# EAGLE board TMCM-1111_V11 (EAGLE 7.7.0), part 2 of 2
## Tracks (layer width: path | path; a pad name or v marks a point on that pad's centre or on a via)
!4361_RST  (via drill 0.3 pad 0.8)
  Top 0.2: IC201.39 41.85,34.05 v40.55,35.35 | IC101.77 31.05,10.75 30.45,11.35 v30.05,11.35
  Bottom 0.2: v30.05,11.35 29.65,11.75 29.65,15.7 29.95,16 30.85,16 32.15,17.3 32.15,24.7 34.65,27.25 34.65,32.25 34.3,32.6 34.3,34.65 34.65,35 36.9,35 37.25,35.35 v40.55,35.35
!CS_262  (via drill 0.3 pad 0.8)
  Top 0.2: IC201.30 48.4,29.75 v48.85,30.2 | IC301.14 v51.26,26.81 v51.25,26.8
  Bottom 0.2: v51.25,26.8 48.85,29.2 v48.85,30.2
!CS_4361  (via drill 0.3 pad 0.8)
  Top 0.2: IC101.5 v32.91,13.29 v32.9,13.3 | IC201.2 39.15,29.25 v38.8,28.9
  Bottom 0.2: v32.9,13.3 v32.89,13.3 v32.9,13.29 34.31,14.7 38.6,14.7 39.45,13.85 41.25,13.85 41.7,14.3 41.7,16.2 44.8,19.3 44.8,20.15 44.1,20.85 44.1,23.25 43.75,23.6 42.5,23.6 40.7,25.4 38.6,25.4 38.15,25.85 38.15,28.25 v38.8,28.9
!CS_EEPROM  (via drill 0.3 pad 0.8)
  Top 0.2: IC503.1 10.92,4.88 v10.9,4.9 | IC101.61 22.9,9.3 v22.2,9.3
  Bottom 0.2: v10.9,4.9 15.7,4.9 16,5.2 16,6.2 18.2,8.4 21.3,8.4 v22.2,9.3
!EN_262  (via drill 0.3 pad 0.8)
  Top 0.2: IC301.15 51.71,26.31 51.45,26.05 50.7,26.05 v50.2,26.55 | IC101.75 30.05,8.35 30.5,7.9 31.5,7.9 32.1,7.3 v32.1,6
  Bottom 0.2: v32.1,6 33.15,7.05 41.45,7.05 43.5,9.1 46.1,9.1 49.85,12.85 49.85,24.7 50.5,25.35 50.5,26.25 v50.2,26.55
!INT_4361  (via drill 0.3 pad 0.8)
  Top 0.2: IC101.73 29.05,8 v31,6.05 | IC201.33 44.85,30.95 45.2,31.3 47.45,31.3 v47.75,31 | LED201.C 46.1,10.04 v46.1,10.7
  Bottom 0.2: v31,6.05 32.35,7.4 38.65,7.4 39.65,8.4 41.7,8.4 43.1,9.8 45.2,9.8 v46.1,10.7 49.15,13.75 49.15,26.4 48.15,27.4 48.15,28.15 47.7,28.6 47.7,30.95 v47.75,31
+3V3  (via drill 0.3 pad 0.8)
  Top 0.2: R501.P$6 34.1,25.4 | 34.1,25.4 33.9,25.6 33.9,26 34.1,26.2 | R501.P$7 34.1,26.2 | 34.1,26.2 33.9,26.4 33.9,26.8 34.1,27 R501.P$8 | IC503.3 13.46,4.84 12.2,6.1 IC503.7 12.19,6.09 12.1,6 11,6 10.9,6.1 10.9,7.2 IC503.8 | 34.1,25.4 33.9,25.2 33.9,24.8 34.1,24.6 R501.P$5 34.9,24.4 v35.75,24.4 | IC203.6 43.05,44.75 42.9,44.9 42.2,44.9 42.05,44.75 IC203.8 | IC201.19 45.35,24.25 45.65,23.95 v46.7,23.95 | IC201.5 40.35,27.75 39.85,27.25 38.75,27.25 38.1,27.9 38.1,28.4 C202.1 | R202.2 41.19,9.81 40.8,10.2 40.8,10.75 39.95,11.6 v39.45,11.6 | IC201.26 v47.5,27.75
  Top 0.25: IC101.50 20.09,16.29 19.9,16.1 19.49,16.1 C104.1 | IC101.70 27.55,8.25 27.9,7.9 27.9,7.45 C102.1
  Top 0.3: IC101.38 24.05,24.53 C105.1 | IC101.7 35.31,14.29 35.6,14 35.6,13.2 35.8,13 36.35,13 C106.1 | IC101.60 20.13,11.23 19.9,11 19.43,11 C103.1 | IC202.8 38.05,43.7 37.9,43.55 C209.2 | IC203.8 42.05,43.75 41.85,43.55 C212.2 | C201.1 44.85,33.35 44.25,33.35 42.85,31.95 IC201.37
  Top 0.5: v24.51,25.93 24.45,25.93 C105.1 26.13,24.93 C408.1 26.34,24.84 26.6,25.1 26.8,25.1 27.1,25.4 28.2,25.4 29.1,24.6 29.5,24.6 29.56,24.46 IC402.5 29.59,24.35 | C106.1 36.95,12.35 36.95,11.6 v37,11.6 | C104.1 18.9,15.6 18.9,15.1 v18.4,14.6 | C102.1 28.45,6.85 28.5,6.8 v28.5,6 | C103.1 19.12,10.42 19.1,10.4 v20.4,10.4 | C503.1 9.35,7.22 IC503.8 9.48,7.22 9.4,7.3 v9.4,8.3 | L101.1 39.8,20 v40.5,20 | C202.1 37.7,28.4 37.45,28.15 36.8,28.15 v36.75,28.1 | C212.2 v40.9,44.6 | C209.2 v36.9,44.6 | v43.6,33.9 44.65,33.9 C201.1 | R302.2 v62.36,25.26 v62.35,25.25 | v51.65,19.35 v47.65,19.35
  Bottom 0.5: TP4.TP 30.71,14.02 v30.7,13.2 | v43.6,33.9 44.5,34.8 44.5,43.65 43.55,44.6 v40.9,44.6 v36.9,44.6 | v62.35,25.25 61.95,25.65 59.4,25.65 57.7,23.95 53.85,23.95 51.65,21.75 v51.65,19.35
  pour Route15 (rank 3): 26.15,26.7 15.8,26.7 15.8,7.8 13.5,7.8 13.5,8.65 8.8,8.65 8.8,6.55 15.8,6.55 15.8,5.4 38.95,5.4 38.95,10.65 42.1,13.8 42.1,18.1 41.4,18.8 41.4,20.35 44.55,20.35 46.1,18.8 48.1,18.8 48.15,18.85 48.15,30.35 43.95,34.6 40.5,34.6 37.2,31.3 30.75,31.3
+5V  (via drill 0.3 pad 0.8)
  Top 0.2: R403.2 32.1,35.15 31.9,35.15 31.5,34.75 24.05,34.75 23.7,35.1 23.7,35.3 22.3,35.3 L402.2 | R503.2 16.15,7.05 15.9,7.3 15.9,8.7 15.6,9 v14.8,9 | R508.P$5 20.25,47.4 20.1,47.55 19.6,47.55 19.45,47.4 | 19.45,47.4 R508.P$6 | 18.65,47.4 18.8,47.55 19.3,47.55 19.45,47.4 | R508.P$7 18.65,47.4 | 18.65,47.4 v18.25,47.8 | 33.4,32 33.25,31.85 33.25,31.35 33.4,31.2 R201.P$8 | R201.P$6 33.4,32.8 | 33.4,32.8 33.25,32.65 33.25,32.15 33.4,32 | 33.6,33.6 33.4,33.6 33.25,33.45 33.25,32.95 33.4,32.8 | R201.P$5 33.6,33.6 | 33.6,33.6 v33.6,34.35 | R201.P$7 33.4,32 | R401.1
  Top 0.38: IC504.8 12.7,31.32 C509.1 | IC505.8 C510.1 | IC506.8 25.4,30.3 | IC204.8 50.02,43.83 49.8,43.6 48.8,43.6 48.6,43.4 C213.2
  Top 0.5: v10.97,25.83 11.87,25.83 C501.2 11.82,25.32 11.82,24.98 11.56,24.71 11.21,24.71 10.92,24.42 IC501.8 | IC502.3 13.44,9.21 C502.2 v14.8,9 | C509.1 12.65,30 12.65,30.35 12.05,30.35 11.85,30.55 11.85,30.85 v11.5,31.2 | C510.1 18.75,29.8 18.1,29.8 v17.9,29.6 | C511.1 25.4,30.3 v24.35,30.3 | 48.8,43.6 48.6,43.8 v48.6,44.6 | R401.1 41.19,18.49 41.4,18.7 41.4,18.9 v42.1,19.6
  Top 0.7: 18.75,40.2 18.79,40.25 C405.1 21,39.95 22.25,39.95 22.3,39.9 L402.2 | v20.1,38.95 19.94,38.79 D401.1 18.75,40.2 | 18.75,40.2 C406.1
  Bottom 0.5: v48.6,44.6 46.65,44.6 45.65,43.6 45.65,37.15 v48.9,33.9
  Bottom 0.7: JP401.1
  other vias: 51.7,16.9
  pour Route15 (rank 4): 56.25,0.5 4,0.5 arc-90 0.5,4 0.5,50.5 arc-90 4.5,54.5 27.5,54.5 27.5,38 46.05,38 51.55,32.5 56.2,32.5
+5V/1  (via drill 0.3 pad 0.8)
  Top 0.2: IC402.3 27.6,27.08 27.6,27.4 26.8,27.4 26.7,27.5 24.6,27.5 v24.3,27.2
  Top 0.5: C407.1 31,26.6 30.8,26.8 | 30.8,26.8 30.8,27.5 v30.6,27.7 | IC402.1 29.78,26.8 30.8,26.8 | v21.25,36.85 21.25,37.85 D401.3
  Route15 0.5: v30.6,27.7 29.95,26.95 28.1,26.95 27.45,27.6 24.75,27.6 24.35,27.2 v24.3,27.2 23.8,27.2 22.8,28.2 22.8,30.4 24.2,31.8 24.2,35.25 22.6,36.85 v21.25,36.85
/EN_D0  (via drill 0.3 pad 0.8)
  Top 0.2: IC504.1 16.57,31.43 16.6,31.4 16.6,30.9 16.7,30.8 16.7,27.7 16,27 16,25.6 16.3,25.3 16.3,24.5 15.6,23.8 v15.6,22.4 | IC101.51 22.2,15.8 v22.5,16.1
  Bottom 0.2: v22.5,16.1 20.9,17.7 20.9,21 21.1,21.2 21.1,22.2 20.6,22.7 15.9,22.7 v15.6,22.4
/EN_D1  (via drill 0.3 pad 0.8)
  Top 0.2: IC505.1 22.98,31.43 23,31.4 23,26.9 22.7,26.6 22,26.6 21.4,27.2 v17.8,27.2 | v25,15.3 24,15.3 23.6,14.9 23.2,14.9 22.09,13.79 IC101.55
  Bottom 0.2: v25,15.3 25,16.1 24.4,16.7 24.1,16.7 23.4,17.4 23.2,17.4 22.1,18.5 22.1,20.4 22.4,20.7 22.4,21.3 23.3,22.2 23.3,23 22.4,23.9 15.7,23.9 14.9,24.7 14.9,25.4 15.6,26.1 15.6,26.4 16.4,27.2 v17.8,27.2
/EN_D2  (via drill 0.3 pad 0.8)
  Top 0.2: IC506.1 29.38,31.43 29.4,31.4 29.4,29.2 29.8,28.8 v30.3,28.8 | IC101.57 22.11,12.79 22.2,12.7 23.8,12.7 v25.6,14.5
  Bottom 0.2: v30.3,28.8 30.75,28.35 31.1,28.35 31.4,28.05 31.4,27.3 30.7,26.6 29.4,26.6 29.1,26.3 29.1,18.95 28.45,18.3 28.45,16.75 27.75,16.05 27.15,16.05 v25.6,14.5
/EN_U0  (via drill 0.3 pad 0.8)
  Top 0.2: IC101.52 22.99,15.29 v23.5,15.8 | IC504.7 13.43,32.08 v13.7,31.8
  Bottom 0.2: v23.5,15.8 23.5,16.2 23.1,16.6 23,16.6 21.3,18.3 21.3,20.8 21.5,21 21.5,22.4 20.8,23.1 15.5,23.1 14.1,24.5 14.1,25.8 14.5,26.2 14.5,27.5 14,28 14,31.5 v13.7,31.8
/EN_U1  (via drill 0.3 pad 0.8)
  Top 0.2: IC505.7 19.68,32.08 20.15,31.6 v20.15,31.15 | v24.2,14.5 23.4,14.5 22.19,13.29 IC101.56
  Bottom 0.2: v24.2,14.5 24.2,16.1 23.3,17 23.1,17 21.7,18.4 21.7,20.5 22,20.8 22,21.4 22.9,22.3 22.9,22.9 22.3,23.5 15.6,23.5 14.5,24.6 14.5,25.6 15.2,26.3 15.2,26.6 16.5,27.9 18.3,27.9 20.15,29.75 v20.15,31.15
/EN_U2  (via drill 0.3 pad 0.8)
  Top 0.2: IC506.7 26.18,32.08 26.5,31.75 v26.5,31.2 | v25.9,15.8 26.35,15.35 26.35,12.15 27.1,11.4 27.1,10.8 26.55,10.25 IC101.68
  Bottom 0.2: v26.5,31.2 25.9,30.6 25.9,22.2 24.7,21 24.7,18.9 25,18.6 25,17.8 25.1,17.7 25.1,17.1 25,17 25,16.7 v25.9,15.8
AIN  (via drill 0.3 pad 0.8)
  Top 0.2: JP101.9 19.08,51.2 17.1,51.2 16.5,50.6 16.5,48.9 15,47.4 11.8,47.4 11.7,47.5 v8.4,47.5 | R502.2 10.47,30.02 10.45,30 v10.45,31.2
  Bottom 0.2: v8.4,47.5 8.4,32.2 9.4,31.2 v10.45,31.2
AIN0  (via drill 0.3 pad 0.8)
  Top 0.2: R505.2 17.15,14.1 16,14.1 14.7,12.8 | IC101.65 25.05,10.15 25.7,10.8 25.7,11.4 25.2,11.9 23.2,11.9 21,9.7 17.8,9.7 17.6,9.9 17.6,10.1 17.2,10.5 C504.1 17.2,11.1 15.9,11.1 15.1,11.9 15.1,12.4 14.7,12.8 | 14.7,12.8 v9.9,12.8 | R502.1 10.47,28.32 10.45,28.3 v10.45,27.25
  Bottom 0.2: v10.45,27.25 9.9,26.7 v9.9,12.8
AIN1
  Top 0.2: IC101.66 25.55,8.45 25.3,8.2 22.2,8.2 21.65,8.75 C505.1 R506.2 R503.1
AIN2  (via drill 0.3 pad 0.8)
  Top 0.2: IC101.67 26.05,8.15 25.4,7.5 24.95,7.5 C506.1 24.55,6.05 v24.6,6 | R504.1 35.2,42.65 R507.2 v34.1,40.3
  Bottom 0.2: v24.6,6 24.6,8.7 25.7,9.8 25.7,11.5 26,11.8 26.9,11.8 27.7,12.6 28.4,12.6 29.2,13.4 29.2,15.9 29.7,16.4 30.7,16.4 31.8,17.5 31.8,24.9 34.3,27.4 34.3,32 32.45,33.85 32.45,34.35 33.8,35.7 33.8,40 v34.1,40.3
BMA1  (via drill 0.3 pad 0.8)
  Top 0.3: 69.94,48.3 v62.1,48.3 | IC301.5 54.49,31.61 54.3,31.8 54.3,33 55,33.7 v55,34.6
  Top 0.38: X301.1 77.09,34.66 77.09,48.26 v73.91,48.26 T301.3
  Bottom 0.3: v55,34.6 56.9,36.5 56.9,44.9 59.1,47.1 60.1,47.1 61.3,48.3 v62.1,48.3
  other vias: 73.91,45.72 73.91,46.99 73.91,50.8 73.91,49.53 67.18,51.94 72.77,51.94 69.98,51.94 68.58,51.94 71.37,51.94 69.98,44.58 72.77,44.58 71.37,44.58 67.18,44.58 68.58,44.58
  pour Top (isolate 0.254, rank 3, no thermals): 66.8,43.73 66.8,54.5 81,54.5 arc-90 84.5,51 84.5,35.2 76.4,35.2 76.4,43.73
  pour Top (rank 4): 76.4,35.2 76.4,31.5 84.5,31.5 84.5,35.3 76.4,35.3
  pour Bottom: 63.5,52.96 63.5,41.66 75.18,41.66 75.18,52.96
BMA2  (via drill 0.3 pad 0.8)
  Top 0.3: 69.97,34.3 v62.1,34.3 | IC301.4 55,30.06 v55,32.5 | 70,32.9 69.98,32.92 T302.3
  Top 0.38: X301.2 77.45,30.8 70,30.8 | 79,29.2 77.8,28 70,28 70,30.8 | 70,30.8 70,32.9
  Bottom 0.3: v62.1,34.3 62.5,33.9 62.5,33 61.2,31.7 55.3,31.7 55,32 v55,32.5
  other vias: 73.91,34.29 73.91,36.83 73.91,31.75 73.91,33.02 73.91,35.56 72.77,37.97 69.98,37.97 67.18,37.97 68.58,37.97 71.37,37.97 71.37,30.61 72.77,30.61 69.98,30.61 67.18,30.61 68.58,30.61
  pour Top (rank 4, no thermals): 66.8,43.23 66.8,27.7 75.9,27.7 75.9,43.23
  pour Top (rank 4): 75.9,31.1 84.5,31.1 84.5,27.7 75.9,27.7
  pour Bottom: 63.5,41.27 63.5,27.69 75.18,27.69 75.18,41.27
BMB1  (via drill 0.3 pad 0.8)
  Top 0.3: 69.98,20.8 v62,20.8 | IC301.20 54.49,23.37 54.48,23.37 54.48,22.48 v54.1,22.1
  Top 0.38: T303.3 69.98,27 77.75,27 X301.3 77.75,24.5 70,24.5
  Bottom 0.3: v62,20.8 60.9,20.8 60.2,20.1 59.1,20.1 58.3,20.9 56.65,20.9 55.45,22.1 v54.1,22.1
  other vias: 73.91,20.83 73.91,23.37 73.91,18.29 72.77,24.51 69.98,24.51 67.18,24.51 68.58,24.51 71.37,24.51 69.98,17.14 72.77,17.14 71.37,17.14 67.18,17.14 68.58,17.14
  pour Top (rank 4, no thermals): 66.8,27.3 76,27.3 76,11.8 66.8,11.8
  pour Top (rank 4): 76,27.3 76,24.1 84.5,24.1 84.5,27.3
  pour Bottom: 63.5,27.3 63.5,13.97 75.18,13.97 75.18,27.3
BMB2  (via drill 0.3 pad 0.8)
  Top 0.3: T304.3 69.92,6.8 v59.3,6.8 | IC301.21 v54.99,21.21 55,21.5
  Top 0.38: X301.4 77.09,20.34 77.09,6.86 v73.91,6.86 | 70.1,6.86 T304.3
  Top 0.406: 70.1,6.86 v73.91,6.86
  Bottom 0.3: v59.3,6.8 59.3,8.2 54,13.5 54,20.23 v54.99,21.21
  other vias: 73.91,9.4 73.91,4.32 73.91,5.59 73.91,8.13 67.18,10.54 72.77,10.54 69.98,10.54 68.58,10.54 71.37,10.54 71.37,3.17 72.77,3.17 69.98,3.17 68.58,3.17 67.18,3.17
  pour Top (isolate 0.254, rank 3, no thermals): 84.5,19.8 76.4,19.8 76.5,11.3 66.9,11.3 66.85,0.5 81,0.5 arc90 84.5,4
  pour Top (rank 4): 76.4,19.32 76.4,23.6 84.5,23.6 84.5,19.32
  pour Bottom: 63.5,13.59 63.5,1.91 75.18,1.91 75.18,13.59
CAN_RX  (via drill 0.3 pad 0.8)
  Top 0.2: IC101.54 20.29,14.29 20.1,14.1 20.1,13.9 v19.7,13.5 | IC502.4 14.71,10.49 14.8,10.4 v15.6,10.4
  Bottom 0.2: v19.7,13.5 16.6,10.4 v15.6,10.4
CAN_TX  (via drill 0.3 pad 0.8)
  Top 0.2: IC101.53 19.79,14.79 v19.5,14.5 | IC502.1 10.89,10.3 11,10.2 v10,10.2
  Bottom 0.2: v19.5,14.5 19.9,14.5 20.4,14 20.4,13.2 19.9,12.7 19.6,12.7 16.5,9.6 15.3,9.6 14.7,10.2 v10,10.2
CANH
  Top 0.2: SV101.4 5.03,19 7.1,19 8.2,17.9 8.2,14.8 9,14 11.5,14 12.16,14.66 IC502.7
CANL
  Top 0.2: SV101.3 7.8,16.33 7.8,14.6 8.8,13.6 12.5,13.6 13.44,14.54 IC502.6
CLK_TMC  (via drill 0.3 pad 0.8)
  Top 0.2: IC301.16 52.23,25.8 51.75,25.8 51.6,25.65 v49.8,25.65 | IC201.38 42.35,32.45 v42.9,33.1 | v26.4,11.1 26.4,11.4 25.5,12.3 IC101.58 | v25.6,5.7 26.1,5.2 33.8,5.2 34.3,5.7 34.3,7.2 34.85,7.75 v40,7.75
  Bottom 0.2: v40,7.75 41.6,7.75 43.3,9.45 45.9,9.45 49.5,13.05 49.5,25.35 v49.8,25.65 49.5,25.95 49.5,26.6 48.5,27.6 48.5,28.4 48.05,28.85 48.05,30.35 48.45,30.75 48.45,31.3 48.05,31.7 44.85,31.7 43.45,33.1 v42.9,33.1 | v26.4,11.1 26.4,9.7 25.6,8.9 v25.6,5.7
D0  (via drill 0.3 pad 0.8)
  Top 0.2: IC504.2 15.57,32.08 15.4,31.9 15.4,30.9 15.6,30.7 15.6,30.35 R509.1 R510.2 16,28.35 15.6,27.95 v15.6,25 | IC101.43 22.49,19.79 v22.8,20.1
  Bottom 0.2: v22.8,20.1 22.8,21.2 23.7,22.1 23.7,23.1 22.5,24.3 16.3,24.3 v15.6,25
D1  (via drill 0.3 pad 0.8)
  Top 0.2: IC505.2 22.6,32.1 22.05,32.1 21.8,31.85 21.8,30.8 21.9,30.7 21.9,30 R513.1 R514.2 22.15,28.3 22.3,28.3 v22.3,27.3 | IC101.45 22.31,18.79 23,18.1 v23.6,18.1
  Bottom 0.2: v22.3,27.3 23.2,26.4 23.2,24.7 24.5,23.4 24.5,21.8 23.9,21.2 23.9,18.4 v23.6,18.1
D2  (via drill 0.3 pad 0.8)
  Top 0.2: v29.6,28.1 28.95,28.1 R518.2 R517.1 28.3,30 28.3,30.7 28.1,30.9 28.1,31.65 28.45,32 28.93,32 IC506.2 | IC101.47 22.31,17.79 23.1,17 23.8,17 24.1,16.7 24.7,16.7 24.9,16.9 26.3,16.9 26.4,16.8 v27.55,16.8
  Bottom 0.2: v29.6,28.1 28.7,27.2 28.7,19.05 28.1,18.45 28.1,17.35 v27.55,16.8
DIR1  (via drill 0.3 pad 0.8)
  Top 0.2: IC301.30 57.92,28.31 58.36,28.75 58.36,29.26 58.6,29.5 v58.6,30.3 | IC201.23 47.7,26.25 49.35,24.6 50.95,24.6 v51.4,24.15 | IC204.2 50.67,40.08 50.4,39.8 v50,39.8
  Bottom 0.2: v51.4,24.15 52.35,24.15 53.55,25.35 55.75,25.35 58,27.6 58,29.7 v58.6,30.3 57.95,30.95 57.1,30.95 56.8,30.65 53.45,30.65 51.55,32.55 51.55,37.45 52.65,38.55 52.65,40.1 52.25,40.5 51.75,40.5 51.05,39.8 v50,39.8
GND  (via drill 0.3 pad 0.8, 0.5 pad 1, 3.2 pad 6.5)
  Top 0.2: T501.2 23.37,44.56 23.37,44.45 | IC301.1 56.84,30.06 57.2,29.7 57.2,29.35 IC301.32 | IC504.4 17.48,33.38 R512.1 | IC505.4 23.88,33.38 R516.1 | R520.1 30.9,30 30.95,29.95 30.95,29.35 v31.3,29 | C214.2 16.3,44.15 16.3,43.05 15.95,42.7 15.95,42.6 15.52,42.17 v15.52,42.16 | 47.6,42.3 47.75,42.15 47.75,41.65 47.6,41.5 R206.P$1 v47,40.7 | 47.6,42.3 R206.P$2 | R206.P$3 47.6,43.1 | 47.6,43.1 47.75,42.95 47.75,42.45 47.6,42.3 | R206.P$4 47.6,43.9 47.75,43.75 47.75,43.25 47.6,43.1 | C210.2 v45.1,48.4 | C211.2 v46.9,48.4 | IC204.1 50.02,40.83 50,40.8 v48.6,40.8 | IC204.7 50.67,42.17 50.6,42.1 | 43.35,29.55 43.4,29.5 43.4,29.45 | IC201.34 44.35,29.55 44.25,29.45 43.4,29.45 | R205.P$4 43.6,21.25 43.55,21.3 42.85,21.3 42.8,21.25 R205.P$3 42.8,21.3 42,21.3 | R205.P$2 42,21.3 | 42,21.3 41.2,21.3 R205.P$1 39.45,20.9 v39.25,21.1 | IC201.6 40.35,27.25 39.95,26.85 38.65,26.85 38.4,27.1 37.9,27.1 37.9,26.85 | C202.2 37.85,26.7 37.9,26.75 | 33.75,30 33.65,29.9 v33.65,29 | 46.9,27.25 47.05,27.1 48.65,27.1 v49.3,27.75 | 43.4,29.45 43.35,29.45
  Top 0.25: IC101.49 20.11,16.79 19.9,17 19.56,17 C104.2 | IC101.69 27.05,8.25 26.9,8.1 26.9,7.45 C102.2 | IC101.59 20.11,11.79 19.9,12 19.51,12 C103.2 | IC201.6 42.85,27.25 v42.85,26.75 | IC201.36 43.35,29.45 43.35,28.25 | 43.35,28.25 v42.85,28.25 42.85,27.5 | v44.35,28.25 43.35,28.25 | v42.85,26.75 43.35,26.75 | 43.35,26.75 v44.35,26.75 44.35,27.25 IC201.25 46.9,27.25 | v42.85,26.75 42.85,27.5 | 42.85,27.5 IC201.41 | IC201.15 43.35,26.75
  Top 0.3: LED401.C LED101.C LED102.C 45.8,14.06 v45.8,13 45.84,12.96 LED202.C | IC301.28 58.5,27.31 58.96,27.77 59.3,27.77 C302.2 | IC301.1 56.49,30.99 57.3,31.8 59.35,31.8 C304.2 | IC301.13 54.49,27.31 IC301.EXP | X101.4 10.8,38.2 11.3,37.7 v11.3,37.4 | X101.5 10.4,37.4 10.4,37.1 v11.2,36.3 | IC101.39 23.55,23.75 23.1,24.2 23.1,24.58 C105.2 | IC101.19 36.1,20.3 36.25,20.15 C110.2 | IC101.8 35.48,14.79 36.37,13.9 37.3,13.9 38,13.2 38,13.05 C106.2 | IC202.4 39.55,42.1 38.85,42.8 38.15,42.8 37.6,42.25 36.9,42.25 C209.1 | IC203.4 43.55,41.65 43.35,41.85 C212.1 | IC201.36 43.35,31.35 v43.6,31.6
  Top 0.38: v36.4,21.35 35.95,21.35 35.45,20.85 IC101.20 | IC204.4 51.98,41.83 51.7,42.1 50.6,42.1 48.7,42.1 48.6,42 C213.1 | C204.2 39.2,32.1 38.9,31.8 38.9,31.35 v38.6,31.05 38.9,30.75 38.9,30 C205.2 | C206.2 38.9,33.7 38.9,34.25 v38.5,34.65
  Top 0.4: IC504.4 v16.2,34.15 | IC505.4 22.9,33.37 v22.9,34.3 | IC506.4 27.62,33.38 v27.5,33.25
  Top 0.5: D101.2 14.01,39.37 13.48,38.84 13.48,37.79 v13.47,37.78 | R105.2 11.53,46.23 v11.44,46.23 | R108.1 15.41,42.16 v15.52,42.16 | R107.1 14.55,36.3 15.1,36.3 15.45,35.95 v15.45,35.45 | IC501.5 14.73,24.44 14.47,24.7 14.32,24.7 14.11,24.92 14.11,25.3 C501.1 14.05,25.84 13.8,25.84 v13.8,26.8 | X101.M2 4.93,43.45 v4.95,43.46 | X101.M1 4.93,34.55 v4.96,34.58 | X101.M4 6.54,34.55 v6.51,34.58 | X101.M3 6.5,43.45 v6.49,43.46 | 23.37,44.58 23.37,44.45 v23.37,42.8 | T502.2 26.92,44.81 v26.92,46.86 | C304.2 60.44,31.46 v61.2,30.7 | C302.2 60.85,28.16 v60.9,28.2 | C105.2 22.45,25.23 22.45,25.85 22.4,25.9 v22.43,25.93 | C408.2 26.13,26.58 25.91,26.8 v25.25,26.8 | IC402.2 28.6,26.3 29.3,25.6 v29.9,25.6 30.4,25.1 30.7,25.1 30.9,24.9 31,24.9 C407.2 | R518.1 26.9,28.35 C511.2 25.35,28.3 v24.3,28.3 | R514.1 20.5,28.35 C510.2 18.95,28.6 v17.9,28.6 | v11.65,27.2 12.3,27.2 12.65,27.55 12.65,28.4 C509.2 12.75,28.4 R510.1 | C113.1 v17.5,22 | Y101.4 18.5,24.8 17.81,24.8 17.8,24.81 v17.2,25.4 | Y101.2 21.23,22.63 21.25,22.6 v22.2,22.6 | C108.2 C109.2 38.6,14.85 38.6,14.2 v38.3,13.9 38.6,13.6 38.6,13.1 38.35,12.85 C106.2 38.35,11.65 v38.3,11.6 | C111.2 C110.2 36.4,20.35 v36.4,21.35 | C112.1 18.7,26.4 18.51,26.2 v17.9,26.2 | C104.2 19.09,17.4 v18,17.4 | R505.1 17.15,15.9 v16.1,15.9 | C107.2 v17.5,18.3 | C102.2 26.55,5.95 v26.6,6 | C506.2 22.85,6.05 v22.9,6 | C505.2 v20.9,6 | C504.2 15.95,12.35 v15.9,12.3 | C103.2 18.9,12.6 18.9,13 v18.4,13.5 | R506.1 v19.1,6 | IC503.4 14.73,3.13 v14.8,3.2 | C503.2 9.32,4.48 v9.4,4.4 | v10.8,9 C502.1 12.16,9.21 IC502.2 | C101.2 7.89,46.25 v6.75,46.25 | IC401.2 30.25,39.6 29.75,39.1 v29.75,38.6
  Top 0.5: R507.1 C209.1 36.9,41.65 36.85,41.6 36,41.6 v35.9,41.5 | C212.1 v40.9,40.8 | C213.1 v48.6,40.8 | C216.2 30.45,45.35 v30.5,45.4 | C401.2 32.08,45.38 v32.1,45.4 | C208.2 v48.1,21.85 | C303.2 51.63,31.42 52,31.05 v52,30.4 | 37.9,26.85 37.9,26.75 37.9,26.5 38,26.4 38.55,26.4 v38.8,26.15 | C201.2 v47.6,33.7 | C207.2 46.8,32.35 v47.6,32.35
  Top 0.7: C307.2 58.35,47.12 v57.89,47.12 v57.88,47.13 | 59.11,47.1 v59.11,45.94 | v58.02,19.68 v58.01,19.69 59.14,19.69 59.19,19.64 59.22,19.64 59.22,19.57 59.27,19.52 59.27,19.67 59.26,19.68 | C306.2 v59.22,18.28 v59.21,18.27 | v22,42.15 C405.2 C406.2 | v23.05,41.5 D402.A 24.05,42.2 24.8,42.95 28.15,42.95 28.19,42.91 C402.2
  Top 1: K302.2 62.75,15.02 R305.1 | K301.2 62.81,42.52 R303.1
  Bottom 0.5: TP5.TP 28.1,11.04 28.1,10.5 26.6,9 v26.6,6
  other vias: 54.74,27.53 54.74,26.38 54.74,28.73 53.54,27.53 55.94,27.53 4,4 81,4 81,51 4,51
  pour Layer2: 0.5,4 arc90 3.9,0.7 81,0.5 arc90 84.5,4 84.5,51 arc90 81,54.5 4,54.5 arc90 0.5,51
  pour Top (rank 4): 66.4,54.5 4,54.5 arc90 0.5,51 0.5,4 arc90 4,0.5 66.45,0.5
  pour Bottom (rank 2): 0.5,51 0.5,4 arc90 4,0.5 81,0.5 arc90 84.5,4 84.5,51 arc90 81,54.5 4,54.5 arc90
LED1  (via drill 0.3 pad 0.8)
  Top 0.2: 41.5,16.3 41.46,16.26 R101.1 41.19,16.31 40.8,16.7 v40.8,17.3 | IC101.31 27.55,20.9 26.95,20.3 26.95,19.25 27.5,18.7 29.65,18.7 31.1,20.15 31.1,20.7 31.6,21.2 33.1,21.2 33.4,21.5 35.35,21.5 35.9,22.05 37.1,22.05 v37.85,21.3
  Bottom 0.2: v37.85,21.3 37.85,20.25 v40.8,17.3
LED2  (via drill 0.3 pad 0.8)
  Top 0.2: 41.19,14.09 R102.1 41.19,14.11 40.8,14.5 v40.8,15.1 | IC101.6 33.41,13.79 33.1,14.1 v33.1,14.5
  Bottom 0.2: v33.1,14.5 34.1,15.5 40.45,15.5 v40.8,15.1
N$1
  Top 0.3: R301.2 LED301.A
N$2
  Top 0.3: IC301.29 58.07,27.81 58.77,28.52 58.77,29.03 59.11,29.37 59.67,29.37 C304.1
  Top 0.5: C304.1 61.74,29.76 62.4,29.1 62.4,28.2 R302.1
N$3
  Top 0.2: 51.39,29.31 50.86,29.31 50.85,29.3 C303.1
  Top 0.3: IC301.9 51.39,29.31
N$4
  Top 0.3: IC301.24 56.49,24.73 56.48,24.72 57.76,24.72 58.94,23.54 59.3,23.54 C301.2
N$5  (via drill 0.3 pad 0.8)
  Top 0.3: T301.5 62.08,45.98 60.8,44.7 v59.8,44.7 | IC301.2 55.99,31.19 56.8,32 56.8,33.8 v57.6,34.6
  Bottom 0.3: v57.6,34.6 57.6,43.5 58.8,44.7 v59.8,44.7
N$6  (via drill 0.3 pad 0.8)
  Top 0.3: T302.5 61.09,32.01 v59.9,33.2 | IC301.3 55.5,31.4 56,31.9 v56,32.5
  Bottom 0.3: v56,32.5 59.2,32.5 v59.9,33.2
N$7  (via drill 0.3 pad 0.8)
  Top 0.3: T302.2 63.7,35.4 v60.7,35.4 | IC301.7 53.49,31.21 52.8,31.9 v52.8,32.3
  Bottom 0.3: v52.8,32.3 53.75,32.3 54.75,33.3 56.4,33.3 56.7,33 58.3,33 v60.7,35.4
N$8  (via drill 0.3 pad 0.8)
  Top 0.3: T301.2 60.9,49.4 60.5,49.8 v59.8,49.8 | IC301.6 53.99,31.41 53.8,31.6 v53.8,34.6
  Bottom 0.3: v53.8,34.6 56.2,37 56.2,46.9 59.1,49.8 v59.8,49.8
N$9  (via drill 0.3 pad 0.8)
  Top 0.3: T303.5 62.05,18.55 61.8,18.3 v61.8,17.3 | IC301.23 55.99,23.31 56.4,22.9 v57.2,22.9
  Bottom 0.3: v61.8,17.3 62.8,18.3 62.8,23 61.9,23.9 61.05,23.9 60.05,22.9 v57.2,22.9
N$10  (via drill 0.3 pad 0.8)
  Top 0.3: T304.5 60.22,4.58 v60.2,4.6 | IC301.22 55.49,21.86 55.9,21.45 55.9,20.7 v55.5,20.3
  Bottom 0.3: v60.2,4.6 60.2,8.3 54.6,13.9 54.6,19.4 v55.5,20.3
N$11  (via drill 0.3 pad 0.8)
  Top 0.3: T303.2 58.83,21.97 v58.8,22 | IC301.19 53.99,23.69 53.3,23 v53.3,21.3
  Bottom 0.3: v58.8,22 56.25,22 55.4,22.85 53.85,22.85 53.3,22.3 v53.3,21.3
N$12  (via drill 0.3 pad 0.8)
  Top 0.3: T304.2 v58.5,8 | IC301.18 53.49,23.99 52.5,23 52.5,20.9 v53.3,20.1
  Bottom 0.3: v58.5,8 53.3,13.2 v53.3,20.1
N$13
  Top 1: K302.1 62.81,12.48 R306.1
N$14
  Top 1: K301.1 62.81,39.98 R304.1
N$15
  Top 0.3: LED202.A R204.2
N$16
  Top 0.3: R202.1 LED201.A
N$17
  Top 0.5: IC401.4 29.2,40.55 | 29.2,40.55 29.5,40.85 29.5,41.25 30.1,41.85 30.9,41.85 30.95,41.9 30.95,42 30.95,42.43 C402.1 | IC401.5 29.25,39.6 29.5,39.85 29.5,40.3 29.2,40.55
  Top 0.7: L401.2 30.95,42
N$18  (via drill 0.3 pad 0.8)
  Top 0.2: IC101.30 28.05,20.75 27.65,20.35 v27.65,19.5 | v20.6,48.05 20.15,48.5 16.7,48.5 15.25,47.05 15.25,46.9 15,46.65 14.3,46.65 14.31,46.64 R105.1
  Top 0.5: R104.2 R105.1
  Bottom 0.2: v27.65,19.5 27.65,20 27.95,20.3 27.95,21.65 27.65,21.95 27.65,28.35 31.1,31.8 31.1,34.15 33.05,36.1 33.05,38.65 24.95,46.75 21,46.75 20.6,47.15 v20.6,48.05
N$19
  Top 0.3: IC101.11 35.51,16.29 35.8,16 35.8,15.6 36,15.4 36.35,15.4 C109.1
N$20
  Top 0.2: IC201.12 41.85,24.25 41.2,23.6 R205.P$8 R203.P$8
N$21  (via drill 0.3 pad 0.8)
  Top 0.2: IC101.9 33.6,15.3
  Top 0.3: X101.3 10.95,39 v11.05,38.9 11.4,38.55 12.08,38.55 D101.6 12.21,37.65 12.3,37.65 12.3,36.58 R107.2 | 33.6,15.3 31.5,15.3 31.1,14.9 29.2,14.9 28.5,14.2 v28.5,13.9
  Bottom 0.3: v11.05,38.9 11.55,38.9 11.85,39.2 13.7,39.2 14.4,38.5 14.4,36.6 12.4,34.6 12.4,20.7 17.5,15.6 19.8,15.6 23,12.4 26.7,12.4 28.2,13.9 v28.5,13.9
N$22  (via drill 0.3 pad 0.8)
  Top 0.2: IC101.10 33.6,15.8
  Top 0.3: X101.2 10.95,39.8 v11.05,39.9 11.4,40.2 12.09,40.2 D101.4 12.21,41.06 12.3,41.15 12.3,41.85 R108.2 | 33.6,15.8 31.3,15.8 30.9,15.4 29,15.4 28.2,14.6 v27.8,14.6
  Bottom 0.3: v11.05,39.9 11.6,39.9 11.85,39.65 13.9,39.65 14.9,38.65 14.9,36.4 12.9,34.4 12.9,20.9 17.7,16.1 20,16.1 23.2,12.9 26.5,12.9 27.8,14.2 v27.8,14.6
N$23
  Top 0.3: R101.2 LED101.A
N$24
  Top 0.3: R102.2 LED102.A
N$25  (via drill 0.3 pad 0.8)
  Top 0.3: IC201.16 43.85,23.95 44.45,23.35 44.45,22.45 44.7,22.2 44.95,22.2 C208.1
  Top 0.5: C208.1 45.65,21.6 45.65,21.1 46,20.75 v47.25,20.75
N$26
  Top 0.2: IC201.35 43.85,30.85 44.4,31.4 44.4,32.1 C207.1
N$27
  Top 0.3: IC101.12 C108.1 36.7,16.8 37,17.1 37,17.4 37.2,17.6 39.1,17.6 39.4,17.3 39.5,17.3 L102.1
N$30
  Top 0.2: IC201.14 42.85,23.95 42.8,23.9 R205.P$6 42.8,22.3 42.25,21.75 38.45,21.75 37.9,22.3 R203.P$6
N$31
  Top 0.2: IC101.40 22.99,23.29 23,23.3 22.5,23.3 21.7,24.1 21.38,24.1 Y101.3 20.93,26.16 C112.2
N$32
  Top 0.2: IC201.13 42.35,24.05 42,23.7 R205.P$7 42,22.3 41.8,22.1 38.9,22.1 38.7,22.3 R203.P$7
N$33
  Top 0.2: IC101.41 19.4,20.85 C113.2 19.2,22.49 Y101.1
N$34
  Top 0.5: IC401.1 30.65,38.65 30.65,38.2 30.4,37.95 30.4,37.2 C404.1
  Top 0.7: C404.1 C403.1
N$35
  Top 0.5: IC401.6 26.95,38.65 26.9,38.6 L402.1
  Top 0.7: D402.C 26.55,41.5 26.55,40.6 26.9,40.25 26.9,38.7 26.95,38.65 | C403.2 C404.2 26.9,37.2 L402.1
N$36  (via drill 0.3 pad 0.8)
  Top 0.2: IC202.7 38.55,43.7 39.95,42.3 v39.95,39.2 | IC201.40 41.35,32.35 v40.9,32.8
  Bottom 0.2: v39.95,39.2 40,39.2 41.2,38 41.2,33.15 v40.9,32.8
N$37  (via drill 0.3 pad 0.8)
  Top 0.2: IC203.7 v42.55,42.65 | IC201.18 44.85,24.2 45.75,23.3 47.1,23.3 v47.7,23.9
  Bottom 0.2: v42.55,42.65 42.55,39.95 41.9,39.3 41.9,31.8 43.5,30.2 44.4,30.2 46.1,28.5 46.1,27.15 47,26.25 47.75,26.25 48.1,25.9 48.1,24.3 v47.7,23.9
N$38
  Top 0.3: LED401.A R401.2
N$40
  Top 0.2: IC401.3 32.4,40.55 R402.2 32.5,40.05 32.55,40.1 33.2,40.1 33.45,39.85 33.45,37.85 33.2,37.6 32.85,37.6 R403.1
N$42
  cutout Bottom (rank 4): 0.6,44.1 3.1,44.1 3.1,29.3 0.6,29.3
N$43
  cutout Bottom (rank 4): 51.7,54.5 58.5,54.5 58.5,51.9 51.7,51.9
  cutout Route15 (rank 4): 51.7,54.5 58.5,54.5 58.5,51.9 51.7,51.9
  cutout Layer2 (rank 4): 51.7,54.5 58.5,54.5 58.5,51.9 51.7,51.9
  cutout Top (rank 4): 51.7,54.5 58.5,54.5 58.5,51.9 51.7,51.9
N$44  (via drill 0.3 pad 0.8)
  Top 0.2: IC201.20 46.25,24.5 46.55,24.8 48.05,24.8 48.75,24.1 48.75,20.9 47.95,20.1 45.25,20.1 44.3,21.05 44.3,21.5 43.85,21.95 v43.4,21.95 43.4,22.7 R205.P$5 | R203.P$5 37.1,23.3 v35.7,23.3
  Bottom 0.2: v35.7,23.3 39.25,23.3 40.6,21.95 v43.4,21.95
N$45  (via drill 0.3 pad 0.8)
  Top 0.2: IC201.10 40.6,25 40.5,24.9 v40.5,24.6 | v39.95,31.05 40.35,31.45 40.35,32.2 40.15,32.4 40.15,34.5 39.85,34.8 v39.85,36.25 | IC202.5 39.55,43.65 v39.85,43.35
  Bottom 0.2: v40.5,24.6 38.9,24.6 37.75,25.75 37.75,28.85 v39.95,31.05 | v39.85,36.25 39.8,36.2 38.45,36.2 37.2,37.45 37.2,42.85 37.7,43.35 v39.85,43.35
N$46  (via drill 0.3 pad 0.8)
  Top 0.2: JP202.2 41.95,3.81 v41.95,6.5 | IC204.3 51.33,39.67 50.5,38.85 v50,38.85
  Bottom 0.2: v41.95,6.5 44.2,8.75 46.3,8.75 50.2,12.65 50.2,24.55 52,26.35 52,28.95 50.5,30.45 50.5,38.35 v50,38.85
N$47  (via drill 0.3 pad 0.8)
  Top 0.2: IC202.2 v38.55,42.1 | IC201.21 47.1,25.25 v47.4,25.55
  Bottom 0.2: v38.55,42.1 41.55,39.1 41.55,31.65 43.35,29.85 44.25,29.85 45.75,28.35 45.75,26.45 46.65,25.55 v47.4,25.55
N$48  (via drill 0.3 pad 0.8)
  Top 0.2: IC204.6 51.33,43.27 52.5,42.1 52.5,40.3 v52,39.8 | JP202.3 43.2,2.52 v43.2,6.5
  Bottom 0.2: v43.2,6.5 45.1,8.4 46.5,8.4 50.55,12.45 50.55,24.4 52.35,26.2 52.35,29.1 50.85,30.6 50.85,38.65 v52,39.8
N$49  (via drill 0.3 pad 0.8)
  Top 0.2: IC203.5 43.55,43.4 v43.4,43.25 | IC201.17 44.35,24.15 45.6,22.9 v48.1,22.9
  Bottom 0.2: v43.4,43.25 43.4,42.4 42.95,41.95 42.95,39.8 42.25,39.1 42.25,31.95 43.65,30.55 44.55,30.55 46.45,28.65 46.45,27.3 47.15,26.6 47.9,26.6 48.45,26.05 48.45,23.25 v48.1,22.9
N$51
  Top 0.2: IC203.3 43.05,40.6 43.2,40.45 43.85,40.45 44.05,40.65 44.05,42.05 44.3,42.3 | R206.P$7 44.3,42.3 | 44.3,42.3 44.15,42.45 44.15,45.2 44.5,45.55 | JP203.2 45.7,52.48 45.7,50.9 44.1,49.3 44.1,45.9 44.45,45.55 44.5,45.55 | C210.1 44.5,45.55
N$52
  Top 0.2: IC203.1 42.05,40.55 42.5,40.1 44.05,40.1 44.6,40.65 44.6,41.5 R206.P$8 45.8,41.5 46.05,41.75 46.05,45.25 46.3,45.5 46.95,45.5 | C211.1 46.95,45.5 | 46.95,45.5 47,45.5 47.6,45.5 48,45.9 48,50.6 48.26,50.86 JP203.3
N$55
  Top 0.5: T502.3 25.77,46.84 25.77,47.99 25.4,48.35 JP101.13
N$56
  Top 0.5: T501.3 22.5,46.84 22.5,48.02 22.86,48.38 JP101.11
NRESET  (via drill 0.3 pad 0.8)
  Top 0.2: R501.P$2 33.3,26.2 33.5,26.4 v33.5,27.9 | C107.1 19.37,19.37 19.7,19.7 19.8,19.7 20,19.9 20,20.2 20.1,20.3 IC101.42 22,20.3 22.5,20.8 23.2,20.8 23.85,20.15 23.85,18.95 25.1,17.7 25.1,17.5 25.3,17.3 27.1,17.3 27.8,18 30.5,18 v30.9,17.6 30.9,17.1 29.65,15.85 28.7,15.85 28.2,15.35 27.35,15.35 26.8,14.8 26.8,12.9 27.6,12.1 31.5,12.1 v32.25,11.35
  Bottom 0.2: v30.9,17.6 31.3,18 31.3,25.1 33.5,27.3 v33.5,27.9 | 33.1,10.9 33.66,11.46 TP3.TP 33.66,11.85 33.65,11.35 v32.25,11.35
OPENDRAIN_1  (via drill 0.3 pad 0.8)
  Top 0.2: T501.1 21.53,45.41 21.84,45.72 23.42,45.72 v23.7,46 | IC101.35 25.55,21.8 24.65,20.9 24.65,19.65 25.15,19.15 v25.6,19.15
  Bottom 0.2: v25.6,19.15 26.1,19.15 26.4,19.45 26.4,19.75 27.25,20.6 27.25,21.25 26.95,21.55 26.95,28.65 30.3,32 30.3,34.5 32.35,36.55 32.35,38.35 25.6,45.1 24.6,45.1 v23.7,46
OPENDRAIN_2  (via drill 0.3 pad 0.8)
  Top 0.2: IC101.36 25.05,21.8 24.25,21 24.25,19.1 25.3,18.05 v25.8,18.05 | T502.1 24.65,44.8 v24.65,46
  Bottom 0.2: v25.8,18.05 26.75,19 26.75,19.6 27.6,20.45 27.6,21.45 27.3,21.75 27.3,28.5 30.7,31.9 30.7,34.35 32.7,36.35 32.7,38.5 25.7,45.5 25.15,45.5 v24.65,46
PHASE_A  (via drill 0.3 pad 0.8)
  Top 0.2: v20.1,43.4 19.45,44.05 R508.P$3 19.45,45.45 19.2,45.7 16.45,45.7 C214.1 16.1,46.8 v17.1,47.8 | IC101.32 27.05,21.8 26.6,21.35 v26.6,20.9 | IC202.1 v38.05,38.5
  Route15 0.2: v31.3,36.45 33.35,38.5 v38.05,38.5
  Bottom 0.2: JP101.10 19.05,51.23 19.05,49.05 18.5,48.5 17.8,48.5 v17.1,47.8 | 19.7,43.8 v20.1,43.4 21.4,44.7 25.5,44.7 32,38.2 32,37.15 v31.3,36.45 29.9,35.05 29.9,32.1 26.6,28.8 v26.6,20.9
PHASE_B  (via drill 0.3 pad 0.8)
  Top 0.2: IC101.33 26.55,21.8 25.65,20.9 v25.65,20.45 | C215.1 17.2,42.45 17.2,42.95 17.65,43.4 v19,43.4 19,43.8 18.85,43.95 18.85,44.52 R508.P$2 | IC202.3 39.05,40.3 38.7,39.95 v38.7,39.2
  Route15 0.2: v31.3,37.5 32.7,38.9 37.3,38.9 37.6,39.2 v38.7,39.2
  Bottom 0.2: JP101.12 21.59,51.23 21.59,49.44 20.9,48.75 20.1,48.75 19,47.65 v19,43.4 19.75,42.65 20.35,42.65 22,44.3 25.4,44.3 31.3,38.4 v31.3,37.5 29.5,35.7 29.5,32.2 26.25,28.95 26.25,21.8 25.65,21.2 v25.65,20.45
PHASE_Z  (via drill 0.3 pad 0.8)
  Top 0.2: R508.P$4 20.25,45.45 21.35,46.55 v21.35,47.45 21.35,48.1 21.59,48.34 21.59,50.8 21.97,51.18 24.08,51.18 JP101.14 | IC101.34 26.05,21.8 25,20.75 25,20.05 25.25,19.8 26,19.8 26.35,19.45 26.35,18.75 v26.9,18.2 | C216.1 28.75,45.45 v28.8,45.5 | IC202.6 39.05,45.45 v39,45.5
  Bottom 0.2: v26.9,18.2 27.4,18.7 27.8,18.7 28.3,19.2 28.3,21.8 28,22.1 28,28.2 31.5,31.7 31.5,33.95 33.4,35.85 33.4,38.8 28.75,43.45 28.75,45.45 | v21.35,47.45 21.7,47.1 25.15,47.1 26.8,45.45 28.75,45.45 | 38.95,45.45 v39,45.5 38.35,46.15 29.45,46.15 v28.8,45.5 28.75,45.45
POSCOMP  (via drill 0.3 pad 0.8)
  Top 0.2: IC101.74 29.55,8.25 30.7,7.1 v31,7.1 | v42.1,10.8 42,10.8 41.5,11.3 41.5,11.62 R204.1 | IC201.31 v46.85,30.5
  Bottom 0.2: v31,7.1 31.65,7.75 38.5,7.75 39.55,8.8 41.05,8.8 41.75,9.5 41.75,10.4 v42.1,10.8 42.5,10.4 44.85,10.4 48.8,14.35 48.8,26.2 48.05,26.95 47.3,26.95 46.85,27.4 v46.85,30.5
PWM_D0  (via drill 0.3 pad 0.8)
  Top 0.2: R509.2 14.6,30 14.6,32.1 13.97,32.73 IC504.6 10.22,32.73 v10.2,32.7
  Bottom 0.2: JP101.3 12.7,46.2 11.7,45.2 10.8,45.2 9.8,44.2 9.8,33.1 v10.2,32.7
PWM_D1  (via drill 0.3 pad 0.8)
  Top 0.2: R513.2 20.9,30.35 20.9,31.45 19.62,32.73 | IC505.6 19.62,32.73 | 19.62,32.73 20.05,33.15 v20.05,33.33
  Bottom 0.2: JP101.5 15.5,49.7 15.5,45.9 17,44.4 17,41.9 18.2,40.7 18.2,35.6 18.9,34.9 18.9,34.48 v20.05,33.33
PWM_D2  (via drill 0.3 pad 0.8)
  Top 0.2: R517.2 27.1,30 27.2,30.1 27.2,31.9 v26.4,32.7 25.43,32.7 IC506.6
  Bottom 0.2: JP101.7 17,49.18 17,48.8 16.3,48.1 16.3,46.2 17.8,44.7 17.8,42.3 18.9,41.2 18.9,36 20.5,34.4 21.8,34.4 22.65,33.55 25.55,33.55 v26.4,32.7
PWM_U0  (via drill 0.3 pad 0.8)
  Top 0.2: JP101.4 12.7,52.45 11.5,51.25 11.5,49.1 12.4,48.2 v14.7,48.2 | v17.8,34.8 14.45,34.8 | IC504.3 14.97,32.73 14.7,33 14.7,34.55 14.45,34.8 | 14.45,34.8 R511.2
  Bottom 0.2: v17.8,34.8 17.8,40.5 16.6,41.7 16.6,44.1 14.7,46 v14.7,48.2
PWM_U1  (via drill 0.3 pad 0.8)
  Top 0.2: R515.2 21,34.9 21,34.2 21.55,33.65 v21.55,33.2 22.02,32.73 IC505.3
  Bottom 0.2: JP101.6 13.97,51.23 13.97,46.14 16.22,43.89 16.22,41.52 17.1,40.64 17.1,34.5 17.55,34.05 18.25,34.05 19.8,32.5 20.35,32.5 21.05,33.2 v21.55,33.2
PWM_U2  (via drill 0.3 pad 0.8)
  Top 0.2: R519.2 30.2,32.05 30.2,32.3 29.77,32.73 IC506.3 28.23,32.73 v27.85,32.35
  Bottom 0.2: JP101.8 16.5,51.22 16.5,48.9 15.9,48.3 15.9,46.1 17.4,44.6 17.4,42.1 18.55,40.95 18.55,35.8 20.3,34.05 21.65,34.05 22.55,33.15 24.95,33.15 26.1,32 27.5,32 v27.85,32.35
REF1  (via drill 0.3 pad 0.8)
  Top 0.2: R203.P$1 39.5,24.2 39.8,23.9 40.05,23.9 v40.3,23.65 | C206.1 37.45,33.6 36.4,33.6 36.35,33.65 | R201.P$4 36.35,33.6 36.35,33.65 | 36.35,33.65 v36.35,34.35 | v31.4,3.75 30.35,4.8 22.62,4.8 20.32,2.5 JP201.2
  Bottom 0.2: v40.3,23.65 40.05,23.9 39,23.9 36.85,26.05 36.85,27 35.45,28.4 35.45,33.45 v36.35,34.35 | 36.35,33.5 v36.35,34.35 | v36.35,34.35 37.3,33.4 39.3,33.4 41.7,30.95 41.7,26.95 43.2,25.45 44.5,25.45 45.95,24 45.95,21.6 46.6,20.95 46.6,18.6 43.6,15.6 43.6,13.45 41.4,11.25 41.4,9.7 40.85,9.15 39.4,9.15 38.35,8.1 31,8.1 30.05,7.15 30.05,5.1 v31.4,3.75
REF2  (via drill 0.3 pad 0.8)
  Top 0.2: JP201.4 26.7,3.75 v29.25,3.75 | v35.8,25.4 36.5,24.7 36.5,24.2 36.7,24 38.5,24 38.7,24.2 R203.P$2 | C204.1 37.55,32.5 36.9,32.5 36.6,32.8 R201.P$3 35.95,32.75 35.9,32.8 35.3,32.8 35.05,33.05 v35.05,34.35
  Bottom 0.2: v29.25,3.75 29.25,8.5 31.35,10.6 31.35,12.8 32.15,13.6 32.15,16.25 32.85,16.95 32.85,24.3 33.95,25.4 v35.8,25.4 36.5,26.1 36.5,26.8 35.05,28.25 v35.05,34.35
REFR1  (via drill 0.3 pad 0.8)
  Top 0.2: R203.P$3 37.7,25.1 37.7,25.5 37.55,25.65 37.25,25.65 36.55,26.35 36.55,27.3 35.8,28.05 35.8,28.55 v36.15,28.9 36.75,28.9 37.1,29.25 37.1,29.6 37.5,30 C205.1 37.1,30 37.1,30.95 36.85,31.2 R201.P$1 | v30.4,3.75 29.75,4.4 24.76,4.4 22.86,2.5 JP201.3
  Bottom 0.2: v36.15,28.9 36.15,29.8 38.2,31.85 40.25,31.85 41.35,30.75 41.35,26.8 43.05,25.1 44.35,25.1 45.6,23.85 45.6,21.45 46.25,20.8 46.25,18.75 43.25,15.75 43.25,13.6 41.05,11.4 41.05,9.9 40.65,9.5 39.25,9.5 38.2,8.45 30.85,8.45 29.7,7.3 29.7,4.45 v30.4,3.75
REFR2  (via drill 0.3 pad 0.8)
  Top 0.2: R203.P$4 36.9,25.05 36.9,25.45 v35.8,26.55 35.8,27.4 35.3,27.9 35.3,30 | 35.3,30 C203.1 | R201.P$2 35.2,32 34.95,31.75 34.95,30.9 35.3,30.55 35.3,30
  Bottom 0.2: JP201.5 27.95,2.53 27.95,4.05 27.55,4.45 27.55,8.4 28.85,9.7 29.85,9.7 30.95,10.8 30.95,11.85 30.05,12.75 30.05,15.4 30.25,15.6 31,15.6 32.5,17.1 32.5,24.5 34.15,26.15 35.4,26.15 v35.8,26.55
RS485+
  Top 0.2: IC501.6 13.46,22.36 13.1,22 13.1,21.3 12.5,20.7 10.1,20.7 9.3,21.5 5,21.5 SV101.6
RS485-
  Top 0.2: IC501.7 12.19,22.49 12.7,22 12.7,21.5 12.3,21.1 10.2,21.1 9.4,21.9 7.2,21.9 6.35,22.75 SV101.7
RS485_DIR  (via drill 0.3 pad 0.8)
  Top 0.2: IC101.37 24.55,21.85 24.2,21.5 20.6,21.5 v20.3,21.8 | IC501.2 12.19,18.99 12.4,19.2 13.3,19.2 13.5,19 13.5,18.11 IC501.3 13.46,18.96 15.1,20.6 15.4,20.6 v15.9,21.1
  Bottom 0.2: v20.3,21.8 19.6,21.1 v15.9,21.1
RS485_RX  (via drill 0.3 pad 0.8)
  Top 0.2: IC101.27 29.55,21.45 29.7,21.3 v30.15,21.3 | IC501.1 10.92,19.12 11.5,19.7 12.7,19.7 v14,21
  Bottom 0.2: v30.15,21.3 30.5,20.95 30.5,19.3 29.2,18 29.2,16.45 28.1,15.35 27.55,15.35 27.1,14.9 27.1,14.4 26.1,13.4 23.7,13.4 17.8,19.3 15.7,19.3 v14,21
RS485_TX  (via drill 0.3 pad 0.8)
  Top 0.2: IC501.4 14.71,18.09 | IC501.4 14.73,17.43 14.7,17.4 15.2,17.4 15.4,17.2 15.4,15 | IC101.28 29.05,21.15 v29.8,20.4 | IC501.4 14.73,18.93 v15.9,20.1
  Bottom 0.2: v29.8,20.4 29.8,19.1 28.85,18.15 28.85,16.6 27.95,15.7 27.4,15.7 26.7,15 26.7,14.5 26,13.8 23.8,13.8 17.9,19.7 16.3,19.7 v15.9,20.1
SCK_DRV  (via drill 0.3 pad 0.8)
  Top 0.2: IC201.29 49.3,29.25 v49.7,29.65 | IC301.12 51.24,27.81 v51.2,27.85
  Bottom 0.2: v49.7,29.65 49.75,29.6 50.45,29.6 51.2,28.85 v51.2,27.85
SDI_DRV
  Top 0.2: IC201.28 46.9,28.75 47,28.85 51.65,28.85 51.69,28.81 IC301.10
SDO_DRV
  Top 0.2: IC201.27 46.95,28.25 47.2,28.5 51.5,28.5 51.69,28.31 IC301.11
SG_TST  (via drill 0.3 pad 0.8)
  Top 0.2: IC301.27 57.97,26.81 v58.32,26.46 | IC101.76 30.55,8.45 30.7,8.3 31.7,8.3 33.15,6.85 v33.15,6 | R301.1 40.8,7.23 v40.8,6.35
  Bottom 0.2: v58.32,26.46 56.86,25 53.75,25 52.15,23.4 51.65,23.4 50.95,22.7 50.95,12.3 46.7,8.05 45.75,8.05 43.5,5.8 41.35,5.8 v40.8,6.35 40.45,6 v33.15,6
SPI0_MISO  (via drill 0.3 pad 0.8)
  Top 0.2: IC101.64 24.55,10.65 v25,11.1 | IC503.2 v12.19,3.99 v12.2,4
  Bottom 0.2: v12.2,4 12.7,4.5 15.9,4.5 16.4,5 16.4,6 18.4,8 22,8 23.4,9.4 23.95,9.4 24.55,10 24.55,10.65 v25,11.1
SPI0_MOSI  (via drill 0.3 pad 0.8)
  Top 0.2: IC101.63 24.05,11.15 v24,11.2 | IC503.5 14.73,6.17 v15.3,5.6
  Bottom 0.2: v15.3,5.6 15.3,6.2 18.1,9 18.7,9 20.9,9 22,10.1 22.8,10.1 23,9.9 23.45,9.9 24.05,10.5 24.05,11.15 v24,11.2
SPI0_SCK  (via drill 0.3 pad 0.8)
  Top 0.2: IC101.62 23.55,10.35 v23.1,10.8 | IC503.6 13.46,6.14 v14,5.6
  Bottom 0.2: v23.1,10.8 22.1,10.8 20.7,9.4 17.8,9.4 v14,5.6
SPI1_MISO  (via drill 0.3 pad 0.8)
  Top 0.2: IC101.4 33.39,12.79 33.2,12.6 v32.2,12.6 | IC201.7 40.4,26.75 v39.85,26.2
  Bottom 0.2: v32.2,12.6 33.21,12.6 33.41,12.8 33.41,12.81 33.8,13.2 41.2,13.2 42.1,14.1 42.1,16.1 45.2,19.2 45.2,20.3 44.45,21.05 44.45,23.45 43.9,24 42.65,24 40.45,26.2 v39.85,26.2
SPI1_MOSI  (via drill 0.3 pad 0.8)
  Top 0.2: IC101.2 33.59,11.79 33.3,11.5 33.3,10.3 v33.6,10 | IC201.4 40.35,28.25 40.05,27.95 v39.05,27.95
  Bottom 0.2: v33.6,10 34.1,10 35,10.9 35,11.8 36,12.8 41.4,12.8 42.5,13.9 42.5,16 45.55,19.05 45.55,20.45 44.8,21.2 44.8,23.6 44.05,24.35 42.8,24.35 42.7,24.45 40.6,26.55 40.6,27.05 39.7,27.95 v39.05,27.95
SPI1_SCK  (via drill 0.3 pad 0.8)
  Top 0.2: IC101.3 35.6,12.3 35.9,12 v35.9,11.6 | IC201.3 40.25,28.75 40.1,28.6 v39.75,28.6
  Bottom 0.2: v39.75,28.6 41,27.35 41,26.65 42.9,24.75 44.2,24.75 45.2,23.75 45.2,21.3 45.9,20.6 45.9,18.9 42.9,15.9 42.9,13.75 41.55,12.4 36.2,12.4 35.9,12.1 v35.9,11.6
SRA  (via drill 0.3 pad 0.8, 0.5 pad 1)
  Top 0.3: IC301.8 52.99,31.01 52.05,31.95 52.05,32.55 v52.8,33.3
  Top 0.7: v61.38,50.54 T301.1 v65.88,50.54 | v61.38,36.57 T302.1 v65.91,36.57 v65.92,36.56 | v67.37,43.22 66.36,43.22 R303.2 66.36,42.12 v67.36,42.12 | v67.35,40.66 66.34,40.66 R304.2 66.36,39.59 v67.36,39.59
  Bottom 0.3: v52.8,33.3 54,33.3 54.5,33.8 56.6,33.8 56.9,33.5 58.1,33.5 59.9,35.3 59.9,36.8 62.69,39.59 v67.36,39.59
  pour Route15: 60.5,51.5 68.5,51.5 68.5,39 68.5,35.5 60.5,35.5 60.5,38.5 61.5,38.5 61.5,48 60.5,48
SRB  (via drill 0.3 pad 0.8, 0.5 pad 1)
  Top 0.3: IC301.17 52.99,24.19 52,23.2 52,20.3 53,19.3 v55.5,19.3
  Top 0.7: v61.47,23.08 63.71,23.09 T303.1 63.74,23.09 v65.92,23.09 | v67.37,15.79 66.36,15.79 R305.2 66.36,14.69 v67.37,14.69 | v67.37,12.86 66.35,12.86 R306.2 66.36,11.77 v67.38,11.77 | v61.35,9.13 63.74,9.12 T304.1 v65.91,9.13
  Bottom 0.3: v67.37,15.79 61.51,15.79 60.8,16.5 56.3,16.5 55.5,17.3 v55.5,19.3
  pour Route15: 60.5,24.5 68.5,24.5 68.5,8 60.5,8 60.5,11.5 61.5,11.5 61.5,21 60.5,21
STEP1  (via drill 0.3 pad 0.8)
  Top 0.2: IC301.31 57.83,28.81 58.01,28.98 58.01,29.89 v57.6,30.3 | IC204.5 51.98,43.23 52.9,42.3 52.9,39.75 v52,38.85 | IC201.24 47.75,26.75 49.55,24.95 v52.15,24.95
  Bottom 0.2: v52.15,24.95 52.9,25.7 55.6,25.7 57.6,27.7 v57.6,30.3 53.25,30.3 51.2,32.35 51.2,38.05 v52,38.85
SWCLK  (via drill 0.3 pad 0.8)
  Top 0.2: IC101.26 30.05,23.55 30.3,23.8 32.1,23.8 32.3,24 32.3,24.5 | 32.4,24.6 32.3,24.6 32.3,24.5 | 32.3,24.5 32.4,24.6 | 32.4,24.6 R501.P$4 33.1,24.6 33.1,23.6 33.5,23.2 v34.2,23.2 | v44.1,19.9 44.45,19.55 46.5,19.55 47.7,18.35 v47.7,17.3
  Bottom 0.2: v34.2,23.2 34.8,22.6 39.35,22.6 40.5,21.45 42.55,21.45 v44.1,19.9 | TP1.TP 47,15.17 47,16.6 v47.7,17.3
SWDIO  (via drill 0.3 pad 0.8)
  Top 0.2: R501.P$3 33.3,25.4 33.5,25.2 33.5,24.3 33.9,23.9 34.5,23.9 34.95,23.45 34.95,22.95 v34.2,22.2 33.5,22.2 32.9,21.6 31.4,21.6 30.7,20.9 30.7,20.25 30.2,19.75 29.5,19.75 28.7,20.55 28.7,21.7 28.55,21.85 IC101.29 | v43.1,19.6 43.5,19.2 46.3,19.2 46.6,18.9 v46.6,17.3
  Bottom 0.2: v34.2,22.2 39.2,22.2 40.3,21.1 42.35,21.1 43.1,20.35 v43.1,19.6 | 43.8,12.1 43.81,12.09 TP2.TP 44.1,11.8 44.1,15.5 45.9,17.3 v46.6,17.3
U0  (via drill 0.3 pad 0.8)
  Top 0.2: v13.7,33.7 13.38,33.38 IC504.5 12.6,34.85 R511.1 | R512.2 17.2,31.5 17.2,30.7 v17.4,30.5 17.1,30.2 17.1,27.5 16.7,27.1 v16.7,26.5 | IC101.44 22.79,19.29 v23.1,19
  Bottom 0.2: v13.7,33.7 14.7,33.7 17.4,31 v17.4,30.5 | v23.1,19 23.5,19.4 23.5,21.4 24.1,22 24.1,23.3 22.7,24.7 16.9,24.7 16.3,25.3 16.3,26.1 v16.7,26.5
U1  (via drill 0.3 pad 0.8)
  Top 0.2: R515.1 19,34.85 IC505.5 19.38,33.38 19.4,33.4 19.4,33.7 19.7,34 20.4,34 20.75,33.65 20.75,32.6 v21.2,32.15 | R516.2 23.65,31.55 23.6,31.5 23.6,30.7 23.4,30.5 23.4,29.6 v23.8,29.2 | IC101.46 22.31,18.29 23.2,17.4 v24.4,17.4
  Bottom 0.2: v24.4,17.4 24.4,18.3 24.3,18.4 24.3,21.1 24.9,21.7 24.9,23.5 23.6,24.8 23.6,26.6 23.4,26.8 23.4,28.8 v23.8,29.2 21.2,31.8 v21.2,32.15
U2  (via drill 0.3 pad 0.8)
  Top 0.2: IC506.5 26.68,33.38 27.2,33.9 30.4,33.9 31.9,32.4 31.9,32.05 R519.1 R520.2 32.05,29.8 v32.05,27.95 | IC101.48 21.19,17.29 21.2,17.3 22.3,17.3 23,16.6 23.7,16.6 24,16.3 24.8,16.3 25,16.5 26.2,16.5 26.6,16.1 28.35,16.1 28.6,16.35 29.15,16.35 v29.9,17.1
  Bottom 0.2: v29.9,17.1 29.9,18.2 30.9,19.2 30.9,25.3 32.05,26.45 v32.05,27.95
USB_VB
  Top 0.5: R103.2 18.69,36.95 D401.2
USB_VBUS  (via drill 0.3 pad 0.8)
  Top 0.3: L102.2 v39.7,14.6 | v32.5,32.85 31,34.35 26.55,34.35 v26.3,34.1 | v20.4,36 16.25,36 15.9,36.35 15.9,38.15 16.05,38.3 16.8,38.3 R103.1
  Top 0.5: X101.1 10.28,40.6 10.29,40.6 10.29,41.08 10.7,41.49 10.9,41.49 11.37,41.96 11.37,44.14 v11.38,44.15 | D101.5 12.23,39.38 12.92,39.38 13.46,39.92 v13.46,40.9 | R104.1 12.57,44.15 v11.38,44.15 | v11.38,44.15 11.38,44.46 11.4,44.48 11.4,45.05 10.45,46 9.85,46 9.62,46.23 C101.1 | 13.44,40.89 v13.46,40.9 | v13.46,40.9 13.66,41.1 15.45,41.1 15.8,40.75 15.8,39.15 16.05,38.9 16.75,38.9 16.8,38.85 R103.1
  Route15 0.3: v39.7,14.6 32.75,21.55 v32.75,28.6
  Bottom 0.3: v32.75,28.6 32.75,30.35 32.5,30.6 v32.5,32.85 | v26.3,34.1 24.8,34.1 22.9,36 v20.4,36
  Bottom 0.5: v11.38,44.15 12.62,44.15 13.46,43.31 v13.46,40.9
V+  (via drill 0.3 pad 0.8, 0.5 pad 1)
  Top 0.3: IC301.25 57.83,25.81 58.05,25.59 58.57,25.59 59.04,26.06 59.3,26.06 C302.1
  Top 0.5: v60.9,24.85 C301.1 C302.1 v60.9,26.45
  Top 0.7: C307.1 60.81,47.1 | 60.81,47.1 v60.81,45.93 | 60.81,47.1 60.83,47.11 | 60.83,47.11 60.83,47.82 60.21,48.44 v59.63,48.44 | 60.83,47.11 60.83,47.12 T301.4 | v65.93,33.16 65.87,33.15 T302.4 61.63,33.15 v61.4,33.15 | v59.59,21.04 60.44,21.04 60.92,20.56 C306.1 | T303.4 C306.1 | 61.36,5.72 v61.34,5.7 63.69,5.7 63.7,5.69 | T304.4 v65.88,5.72 | C306.1 60.92,18.32 | L401.1 33.92,44.27 C401.1 35.24,44.41 R504.2 35.3,44.45 v35.3,45.5
  other vias: 60.9,18.3
  pour Route15 (rank 2): 28,54.5 81,54.5 arc-90 84.5,51 84.5,4 arc-90 81.1,0.5 56.55,0.5 56.5,32.8 51.7,32.8 46.2,38.3 28,38.3
VDDA
  Top 0.3: IC101.18 35.51,19.79 35.7,19.6 35.7,19.5 35.5,19.3 | IC101.17 35.49,19.29 35.5,19.3 | 35.5,19.3 35.5,19.2 35.9,18.8 36.25,18.8 C110.1
  Top 0.5: C110.1 C111.1 39.65,18.45 L101.2

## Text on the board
Top: 1 | Top Layer 1
Layer2: 2 | Inner Layer 2
Route15: 3 | Inner Layer 3
Bottom: 4 | V11-170802 | Bottom Layer 4
Dimension: TMCM-1111_V11 02.08.2017
tPlace: 2 | 14 | 1 | Step/Dir In | 13 | GPIO | 1A/2.8A | A1 | A2 | B1 | B2 | Power | Silksreen Top | Led 1 | Led 2 | PosComp | 1A/2.8A | RS485/CAN | Interrupt | stallGuard2 | GND | L | R | H | ST | Step/Dir Out | +5V GND | TMCM-1111 V1.1
bPlace: Silksreen Bottom
tStop: Solder Mask Top
bStop: Solder Mask Bottom
tCream: Paste Mask Top
bCream: Paste Mask Bottom
Drills: Drill Drawing
tDocu: Assembly Top
bDocu: Assembly Bottom
DrillLegend: Drill-Drawing
tRef: JP203 | DRILEGEND | H403 | JP101 | H402 | X401 | T301 | C307 | C101 | R105 | R508 | T501 | T502 | C210 | C211 | C214 | R104 | C216 | C401 | R504 | C209 | IC202 | C212 | IC203 | R206 | C213 | IC204 | R303 | R108 | D402 | C402 | L401 | C308 | C215 | C406 | C405 | K301 | IC401 | R402 | R507 | R304 | X101 | D101 | R103 | D401 | L402 | R107 | C404 | C403 | R403 | R511 | R515 | C206 | C201 | T302 | IC504 | R512 | IC505 | R516 | IC506 | R519 | R201 | C204 | C207 | C303 | C304 | R509 | R513 | R517 | R520 | C203 | C205 | R502 | C509 | C510 | C511 | R510 | R514 | R518 | C202 | IC201 | IC301 | X301 | C302 | R302 | C501 | C112 | C408 | IC402 | C407 | R501 | C105 | Y101 | R203 | C301 | R205 | C208 | IC501 | C113 | T303 | SV101 | C306 | C107 | C110 | C111 | L101 | R401 | LED401 | C104 | C108 | IC101 | L102 | R101 | LED101 | R505 | C109 | R305 | R102 | LED102 | K302 | C305 | IC502 | C106 | C504 | C103 | R204 | LED202 | R306 | R202 | LED201 | C502 | R503 | R506 | C505 | R301 | LED301 | C506 | C102 | T304 | C503 | IC503 | H404 | H401 | JP201 | JP202 | JP401
bRef: TP4 | TP1 | TP5 | TP3 | TP2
